TYPE IDENTControl_UserData_IUH_MF :
STRUCT	
	ReadData:			ARRAY[0..245] OF BYTE;	(* Read in data from data carrier*)	
	WriteData:			ARRAY[0..245] OF BYTE;	(* Write data to data carrier *)
	SpecialCommand:		ARRAY[0..30] OF BYTE;	(* Bypass for commands, which are not included in FB *)
	NumberTags:			ARRAY[0..3] OF BYTE;	(* Number of tags identified during Single command; 16#30303031 = 1 Tag; 16#30303030 = 0 Tag*)
	TagInformation:		ARRAY[0..4] OF BYTE;	(* Contains further information about tag access; only transmit if parameter IF = 16#01; Byte 0 = Info Type; Byte 1 = RSSI; Byte 2 = Channel; Byte 3/4 = Output power*)
	EPC_WrittenTag:		ARRAY[0..55] OF BYTE;	(* UII/EPC Code of the successfully written tag*)
	EPC_LeaveTag:		ARRAY[0..55] OF BYTE;	(* UII/EPC Code of the tag which leaves the detection zone during Enhanced command*)
	ReadParam_IF:		BYTE;					(* Parameter IF; information frame with RSSI; only MultiFrame; Default = 16#00; 16#00 = switched off; 16#01 = switched on*)
	ReadParam_AP:		BYTE;					(* Parameter AP; Antenna polarization; Default = 16#43 "C" Combined Mode*)
	ReadParam_CD:		ARRAY[0..3] OF BYTE;	(* Parameter CD; used channels; Default channel 4, 10, 7, 13*)
	ReadParam_E5 : 		BYTE;					(* Parameter E5; Tag Lost smoothing; Default = 16#05*)
	ReadParam_MB : 		BYTE;					(* Parameter MB; Memory Bank; Default 16#03*)
	ReadParam_NT : 		BYTE;					(* Parameter NT; Number of Tags to find; Default = 16#FF*)
	ReadParam_QV : 		BYTE;					(* Parameter QV; Protocol Mode; Default = 16#4D MultiFrame Protocol*)
	ReadParam_QW : 		BYTE;					(* Parameter QW; Definition of used Time slots; Default = 16#02*)
	ReadParam_SM :		WORD;					(* Parameter SM; Sensing Mode; Default 16#0064*)
	ReadParam_TA : 		BYTE;					(* Parameter TA; Tries allowed; Default = 16#02*)
	ReadParam_PT : 		ARRAY[1..10] OF WORD;	(* Parameter PT; Power setting; Default = 16#0032 50mW; depending on connected device type*)
	ReadParam_MF: 		ARRAY[0..51] OF BYTE;	(* Parameter MF; measured reflection of the used channels*)
	ReadParam_RC :		WORD;					(* Parameter RC; Region Code*)
	ReadParam_NC :		BYTE;					(* Parameter NC; number of channels*)
	ReadParam_FL_0 :	ARRAY[0..19] OF BYTE;	(* Parameter FL; filter configuration of filter number 0*)
	ReadParam_FL_1 :	ARRAY[0..19] OF BYTE;	(* Parameter FL; filter configuration of filter number 1*)
	ReadParam_FL_2 :	ARRAY[0..19] OF BYTE;	(* Parameter FL; filter configuration of filter number 2*)
	ReadParam_SE :		BYTE;					(* Parameter SE; Session; Default = 16#01; do not change!!!*)
	ReadParam_FB :		BYTE;					(* Parameter FB; Search Mode; Default = 16#00; do not change!!!*)
	ReadParam_FR :		BYTE;					(* Parameter FR; Sequence Mode; Default 16#00 (Write after Read); do not change!!!*)
	ReadParam_EF :		BYTE;					(* Parameter EF; Fixcode length; Default = 16#00; do not change!!!*)
	
	WriteParam_IF: 		BYTE := 16#00;			(* Parameter IF; information frame with RSSI; only MultiFrame; Default = 16#00; 16#00 = switched off; 16#01 = switched on*)
	WriteParam_AP: 		BYTE := 16#43;			(* Parameter AP; Antenna polarization; Default = 16#43 "C" Combined Mode*)
	Length_CD:			INT := 4;				(* Length of the parameter CT; Default = 4; 4 channels*)
	WriteParam_CD:		ARRAY[0..3] OF BYTE := [16#04, 16#0A, 16#07, 16#0D];			(* Parameter CD; used channels; Default channel 4, 10, 7, 13*)
	WriteParam_E5:		BYTE := 16#05;			(* Parameter E5; Tag Lost smoothing; Default = 16#05*)
	WriteParam_MB:		BYTE := 16#03;			(* Parameter MB; Memory Bank; Default 16#03*)
	WriteParam_NT:		BYTE := 16#FF;			(* Parameter NT; Number of Tags to find; Default = 16#FF*)
	WriteParam_QV:		BYTE := 16#4D;			(* Parameter QV; Protocol Mode; Default = 16#4D MultiFrame Protocol*)
	WriteParam_QW:		BYTE := 16#02;			(* Parameter QW; Definition of used Time slots; Default = 16#02*)
	WriteParam_SM:		WORD := 16#0064;		(* Parameter SM; Sensing Mode; Default 16#0064*)
	WriteParam_TA:		BYTE := 16#02;			(* Parameter TA; Tries allowed; Default = 16#02*)
	Length_PT:			INT := 2;				(* Length of the parameter PT; 2 = 2 Byte; 2 Byte for each power level*)
	WriteParam_PT:		ARRAY[1..10] OF WORD := [16#0032, 16#0000, 16#0000];		(* Parameter PT; Power setting; Default = 16#0032 50mW; depending on connected device type*)
	WriteParam_RC:		WORD := 16#0001;		(* Parameter RC; Region Code*)	
	WriteParam_NC:		BYTE := 16#04;			(* Parameter NC; number of channels*)
	WriteParam_SE:		BYTE := 16#01;			(* Parameter SE; Session; Default = 16#01; do not change!!!*)
	WriteParam_FB:		BYTE := 16#00;			(* Parameter FB; Search Mode; Default = 16#00; do not change!!!*)
	WriteParam_FR:		BYTE := 16#00;			(* Parameter FR; Sequence Mode; Default 16#00 (Write after Read); do not change!!!*)
	WriteParam_EF:		BYTE := 16#00;			(* Parameter EF; Fixcode length; Default = 16#00; do not change!!!*)
END_STRUCT
END_TYPE
